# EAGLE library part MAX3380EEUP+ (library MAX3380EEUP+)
Dual Transmitter/Receiver RS-232 Source: Datasheet
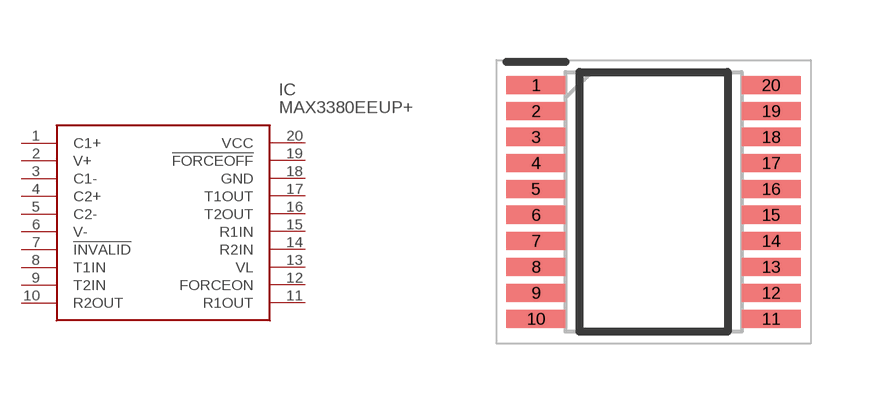
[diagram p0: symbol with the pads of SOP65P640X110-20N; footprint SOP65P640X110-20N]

Designator prefix IC

## MAX3380EEUP+ (Description: Dual Transmitter/Receiver RS-232; Height: 1.1mm; Manufacturer_Name: Maxim Integrated; Manufacturer_Part_Number: MAX3380EEUP+; RS_Part_Number: 7329452P; RS_Price-Stock: http://uk.rs-online.com/web/p/products/7329452P)  [SOP65P640X110-20N]
1  C1+
2  V+
3  C1-
4  C2+
5  C2-
6  V-
7  !INVALID
8  T1IN
9  T2IN
10  R2OUT
11  R1OUT
12  FORCEON
13  VL
14  R2IN
15  R1IN
16  T2OUT
17  T1OUT
18  GND
19  !FORCEOFF
20  VCC

## Footprint SOP65P640X110-20N (pad centres in mm)
MAX3380EEUP+
smd 1.475 x 0.45: 1 -2.938,2.925; 2 -2.938,2.275; 3 -2.938,1.625; 4 -2.938,0.975; 5 -2.938,0.325; 6 -2.938,-0.325; 7 -2.938,-0.975; 8 -2.938,-1.625; 9 -2.938,-2.275; 10 -2.938,-2.925; 11 2.938,-2.925; 12 2.938,-2.275; 13 2.938,-1.625; 14 2.938,-0.975; 15 2.938,-0.325; 16 2.938,0.325; 17 2.938,0.975; 18 2.938,1.625; 19 2.938,2.275; 20 2.938,2.925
